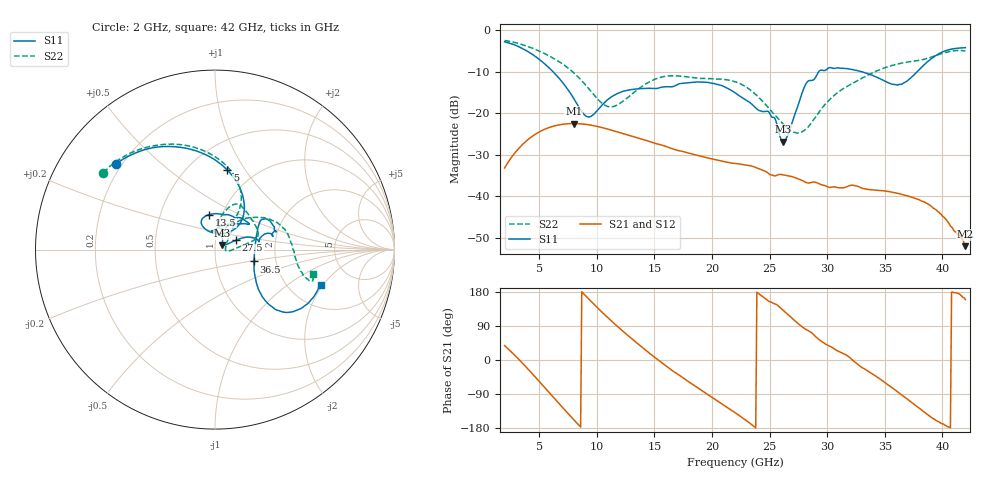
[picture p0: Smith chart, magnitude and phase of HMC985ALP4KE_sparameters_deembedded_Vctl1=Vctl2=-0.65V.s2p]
!s2p File: Measurements: S11, S21, S12, S22
# GHz S dB R 50.0
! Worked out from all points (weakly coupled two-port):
!   401 points, 2 GHz to 42 GHz, reference 50 ohm
!   highest |S21| = -22.44 dB at 8 GHz (marker M1); lowest = -52.0 dB at 42 GHz (marker M2)
!   lowest |S11| = -26.8 dB at 26.2 GHz (marker M3), VSWR 1.10, Z = 54 + j2.61 ohm
!   |S11| at or under -10 dB: 6.218 GHz to 29.26 GHz (23.04 GHz wide, 130 % of centre); 33.06 GHz to 37.8 GHz (4.743 GHz wide, 13.4 % of centre)
!   |S22| runs from -24.8 to -2.4 dB; largest |S21 - S12| = 0.00015
!   S11 on the Smith chart (normalised r, x): 2 GHz: 0.18, +0.36; 5 GHz: 0.75, +0.83; 13.5 GHz: 0.87, +0.35; 27.5 GHz: 1.26, +0.13; 36.5 GHz: 1.53, -0.21; 42 GHz: 2.96, -1.88
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2  -2.74 138.9  -33.16 37.9  -33.16 37.9  -2.43 145.4
3.4  -4.17 112.1  -27.93 -3.5  -27.93 -3.5  -3.33 122.9
5  -6.97 81.1  -24.47 -56.3  -24.47 -56.4  -4.97 98.3
8  -16.41 46.9  -22.44 -157.5  -22.45 -157.5  -10.21 61.8
8.7  -19.59 59.9  -22.54 179.9  -22.54 179.9  -12.14 58.0
9.5  -20.71 92.2  -22.84 154.9  -22.84 154.9  -14.70 57.8
11  -16.57 118.0  -23.82 110.6  -23.83 110.6  -18.37 72.9
13.5  -14.08 100.1  -25.87 44.4  -25.88 44.4  -14.35 79.0
15.4  -13.87 74.1  -27.46 -1.3  -27.46 -1.3  -11.43 68.3
18.9  -12.45 37.8  -30.23 -76.2  -30.24 -76.2  -11.52 40.6
22  -15.02 54.0  -32.07 -138.8  -32.07 -138.7  -12.37 15.5
24.9  -19.54 95.0  -34.44 155.7  -34.45 155.7  -18.63 3.5
26.2  -26.78 31.7  -34.81 130.3  -34.82 130.3  -22.62 -6.5
27.5  -17.80 23.9  -35.79 95.6  -35.79 95.8  -24.69 2.8
28.1  -13.19 18.0  -36.53 81.6  -36.56 81.6  -23.94 18.1
28.7  -12.03 10.7  -36.60 70.5  -36.59 70.2  -22.01 31.8
31  -9.04 21.4  -37.92 22.6  -37.92 22.8  -14.79 51.7
33.3  -10.22 32.7  -38.22 -24.6  -38.23 -24.6  -11.14 40.2
35.4  -12.71 11.3  -38.87 -68.2  -38.89 -68.0  -8.65 24.9
36.5  -12.93 -17.1  -39.55 -92.7  -39.55 -92.9  -7.83 15.9
39.6  -5.80 -42.7  -43.63 -162.2  -43.62 -162.0  -5.91 -15.6
42  -4.16 -18.4  -51.99 159.3  -51.95 158.4  -4.96 -14.1
